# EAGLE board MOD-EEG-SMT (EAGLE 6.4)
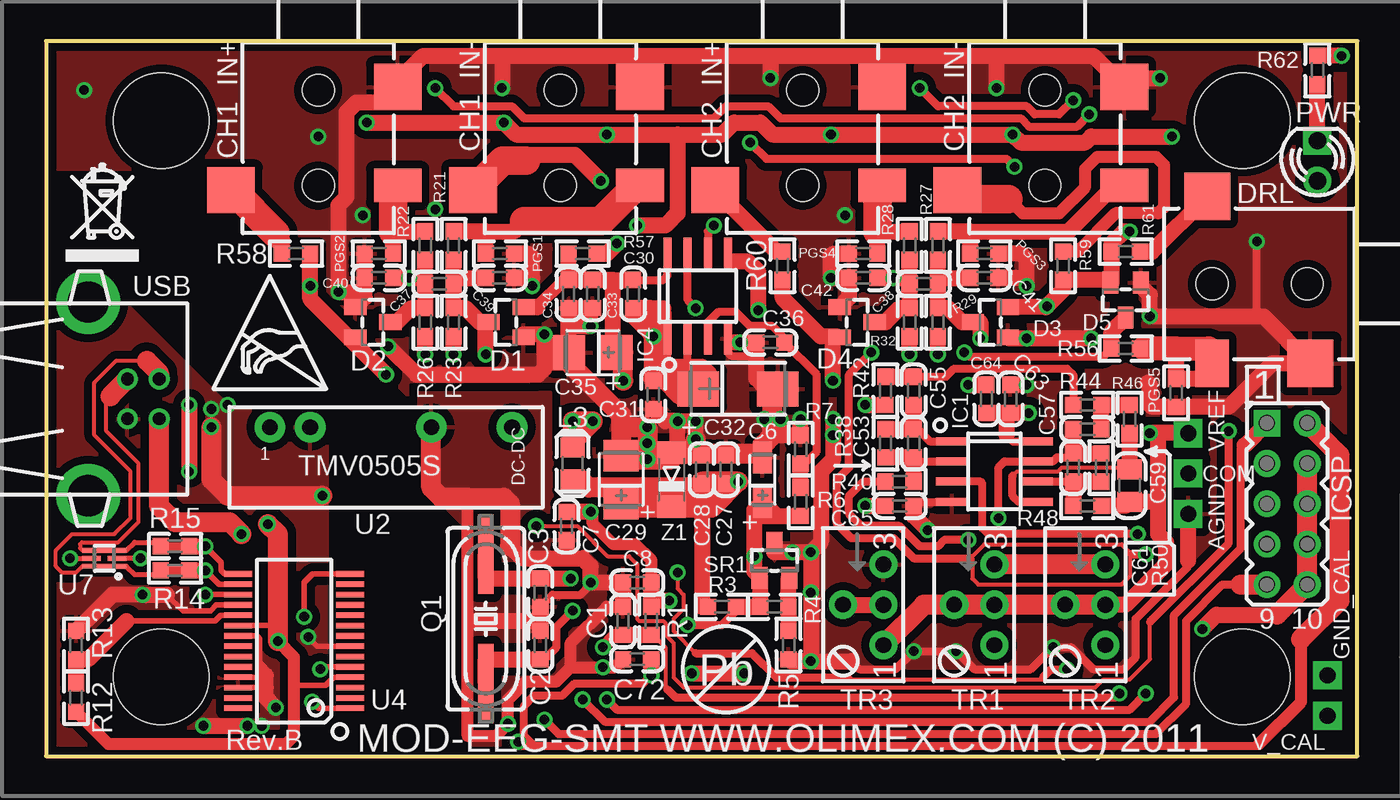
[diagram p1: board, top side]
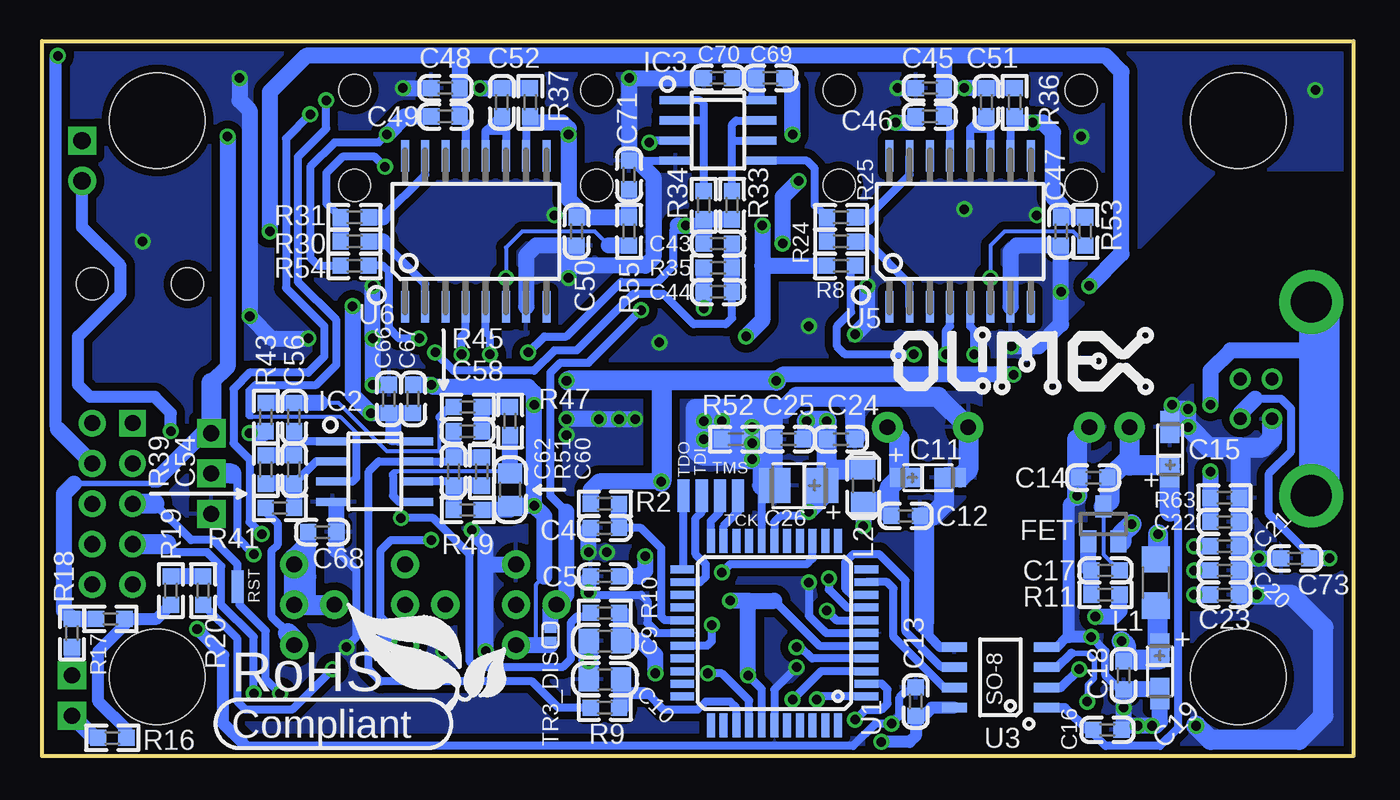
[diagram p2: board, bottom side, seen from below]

Size 82.5 x 45 mm. Coordinates in mm from the lower left corner, seen from the top.
Outline: 0,0 82.5,0 82.5,45 0,45 0,0
Copper layers (1+16): Top 0.035mm / dielectric 1.5mm / Bottom 0.035mm
Design rules "default": minimum track width 10mil, minimum drill 0.5994mm, track to track 10mil, track to pad 10mil, pad to pad 10mil, via to via 10mil, smd to smd 1mil, copper to edge 10mil, drill to drill 10mil, minimum pad ring 10mil, minimum via ring 8mil, stop-mask expansion 4mil, vias tented up to drill 25mil, thermal gap 20mil
Net classes: 1 pwr: width 0.4 mm, clearance 0.23 mm
Holes 6 mm at 7.25,5 75.25,5 7.25,40 75.25,40
tKeepout: area 22.5,43 to 30.5,45; area 21.2,0.2 to 29.2,2.2; area 45.9,0.1 to 61.9,2.1; area 45.3,43 to 61.3,45
bKeepout: area 46.8,43 to 62.8,45; area 22.5,43 to 30.5,45; area 21.2,0.2 to 29.2,2.2; area 47.3,0.2 to 63.3,2.2
tRestrict: 20 lines
bRestrict: 22 lines

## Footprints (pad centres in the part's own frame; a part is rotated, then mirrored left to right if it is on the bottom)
TEST_PAD40/70/SQUARE = drill 1.016 pad 1.778 square: P$1 0,0
C0603_DWS = smd 1.016 x 1.016: 1 -0.889,0; 2 0.889,0
CT3216 = smd 2 x 1.2: + -1.4,0; - 1.4,0
C0805_5MIL_DWS = smd 1.27 x 1.524: 1 -1.016,0; 2 1.016,0
C0603_DWS_NA = smd 1.016 x 1.016: 1 -0.889,0; 2 0.889,0
CT3528 = smd 2 x 2.2: + -1.5,0; - 1.5,0
CT6032 = smd 2.6 x 2.2: + -2.5,0; - 2.5,0
PHONE_JACK-SMD = smd 2.9 x 3: 1 -0.2,5; 5 6.3,-5.5 | smd 2.1 x 3: 2 6,5 | hole 2: 0,0; 6,0
SOT23C(BAT54S) = smd 1 x 1.4: 1 -0.95,-1.1; 2 0.95,-1.1; 3 0,1.1
SOT23 = smd 1 x 1.4: 1 -0.95,-1.1; 2 0.95,-1.1; 3 0,1.1
SO08 = smd 0.508 x 2.032: 1 -1.905,-2.667; 2 -0.635,-2.667; 3 0.635,-2.667; 4 1.905,-2.667; 5 1.905,2.667; 6 0.635,2.667; 7 -0.635,2.667; 8 -1.905,2.667
ML10_NEW = drill 1.016 pad 1.676 square: 1 -5.08,-1.27 | drill 1.016 pad 1.676: 2 -5.08,1.27; 3 -2.54,-1.27; 4 -2.54,1.27; 5 0,-1.27; 6 0,1.27; 7 2.54,-1.27; 8 2.54,1.27; 9 5.08,-1.27; 10 5.08,1.27
L1206_5MIL = smd 1.651 x 1.778: 1 -1.46,0; 2 1.46,0
L0805_5MIL_DWS = smd 1.27 x 1.524: 1 -1.016,0; 2 1.016,0
0603 = smd 1.016 x 1.016: 1 -0.889,0; 2 0.889,0
LED-3.0MM = drill 1.092 pad 1.778: A -1.27,0 | drill 1.092 pad 1.778 square: K 1.27,0
HC49/SMD2_THIN = smd 5 x 1: 1 -4.064,0; 2 4.064,0
R0603_5MIL_DWS = smd 1.016 x 1.016: 1 -0.889,0; 2 0.889,0
R0603_5MIL_DWS_NA = smd 1.016 x 1.016: 1 -0.889,0; 2 0.889,0
0603_0R = smd 1.016 x 1.016: 1 -0.889,0; 2 0.889,0
SMD80/30 = smd 2.032 x 0.762: P$1 0,0
SOT-23 = smd 1 x 1.4: 1 -0.95,-1.1; 2 0.95,-1.1; 3 0,1.1
S64Y = drill 0.991 pad 1.778: 1 2.54,1.27; 2 0,-1.27; 3 -2.54,1.27
SJ_1_SMALLER = smd 0.508 x 0.762: 1 -0.381,0; 2 0.381,0
44TQFP = smd 1.5 x 0.5: 1 -5.8,4; 2 -5.8,3.2; 3 -5.8,2.4; 4 -5.8,1.6; 5 -5.8,0.8; 6 -5.8,0; 7 -5.8,-0.8; 8 -5.8,-1.6; 9 -5.8,-2.4; 10 -5.8,-3.2; 11 -5.8,-4; 23 5.8,-4; 24 5.8,-3.2; 25 5.8,-2.4; 26 5.8,-1.6; 27 5.8,-0.8; 28 5.8,0; 29 5.8,0.8; 30 5.8,1.6; 31 5.8,2.4; 32 5.8,3.2; 33 5.8,4 | smd 0.5 x 1.5: 12 -4,-5.8; 13 -3.2,-5.8; 14 -2.4,-5.8; 15 -1.6,-5.8; 16 -0.8,-5.8; 17 0,-5.8; 18 0.8,-5.8; 19 1.6,-5.8; 20 2.4,-5.8; 21 3.2,-5.8; 22 4,-5.8; 34 4,5.8; 35 3.2,5.8; 36 2.4,5.8; 37 1.6,5.8; 38 0.8,5.8; 39 0,5.8; 40 -0.8,5.8; 41 -1.6,5.8; 42 -2.4,5.8; 43 -3.2,5.8; 44 -4,5.8
TMADCDC = drill 0.991 pad 1.93: 1 1.27,6.35; 2 1.27,3.81; 5 1.27,-3.81; 7 1.27,-8.89
SO-8_ISOLATE = smd 0.6 x 1.6: 1 -1.905,-2.9; 2 -0.635,-2.9; 3 0.635,-2.9; 4 1.905,-2.9; 5 1.905,2.9; 6 0.635,2.9; 7 -0.635,2.9; 8 -1.905,2.9
SSOP28 = smd 0.35 x 1.75: 1 -4.225,-3.525; 2 -3.575,-3.525; 3 -2.925,-3.525; 4 -2.275,-3.525; 5 -1.625,-3.525; 6 -0.975,-3.525; 7 -0.325,-3.525; 8 0.325,-3.525; 9 0.975,-3.525; 10 1.625,-3.525; 11 2.275,-3.525; 12 2.925,-3.525; 13 3.575,-3.525; 14 4.225,-3.525; 15 4.225,3.525; 16 3.575,3.525; 17 2.925,3.525; 18 2.275,3.525; 19 1.625,3.525; 20 0.975,3.525; 21 0.325,3.525; 22 -0.325,3.525; 23 -0.975,3.525; 24 -1.625,3.525; 25 -2.275,3.525; 26 -2.925,3.525; 27 -3.575,3.525; 28 -4.225,3.525
SO16 = smd 0.5 x 2: 1 -4.445,-4.75; 2 -3.175,-4.75; 3 -1.905,-4.75; 4 -0.635,-4.75; 5 0.635,-4.75; 6 1.905,-4.75; 7 3.175,-4.75; 8 4.445,-4.75; 9 4.445,4.75; 10 3.175,4.75; 11 1.905,4.75; 12 0.635,4.75; 13 -0.635,4.75; 14 -1.905,4.75; 15 -3.175,4.75; 16 -4.445,4.75
USBLC6-2P6 = smd 0.3 x 1.46: 1 -0.5,-0.65; 3 0.5,-0.65; 4 0.5,0.65; 6 -0.5,0.65 | smd 0.3 x 1.16: 2 0,-0.8; 5 0,0.8
USB_NEAR_BLACK = drill 0.8: 1 1.25,6.5; 2 -1.25,6.5; 3 -1.25,4.5; 4 1.25,4.5 | drill 2.6 pad 4: P$1 -6.096,2.032; P$2 6.096,2.032
MINI-MELF = smd 1.4 x 1.8: 1 -1.7,0; 2 1.7,0

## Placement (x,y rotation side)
AGND  TESTPAD3  [TEST_PAD40/70/SQUARE]  71.86,15.24 90 top
C1  100nF/X7R/10%  [C0603_DWS]  36.3,8.51 90 top
C2  39pF/COG/5%  [C0603_DWS]  31.09,6.99 90 top
C3  39pF/COG/5%  [C0603_DWS]  31.09,10.29 270 top
C4  10nF/X7R/10%  [C0603_DWS]  47.09,14.35 180 bottom
C5  100nF/X7R/10%  [C0603_DWS]  47.09,11.3 180 bottom
C6  10uF/6.3V/TANT  [CT3216]  45.06,17.4 90 top
C7  100nF/X7R/10%  [C0603_DWS]  32.74,14.48 270 top
C8  100nF/X7R/10%  [C0603_DWS]  37.19,10.92 180 top
C9  220nF/X7R/5%(08053C224JAT2A/1740667)  [C0805_5MIL_DWS]  47.09,7.24 180 bottom
C10  220nF/X7R/5%(08053C224JAT2A/1740667)  [C0805_5MIL_DWS]  47.09,4.83 180 bottom
C11  10uF/6.3V/TANT  [CT3216]  26.77,17.53 0 bottom
C12  100nF/X7R/10%  [C0603_DWS]  28.17,15.11 0 bottom
C13  100nF/X7R/10%  [C0603_DWS]  27.54,3.43 90 bottom
C14  100nF/X7R/10%  [C0603_DWS]  16.36,17.53 180 bottom
C15  10uF/6.3V/TANT  [CT3216]  11.53,19.3 90 bottom
C16  100nF/X7R/10%  [C0603_DWS]  15.47,1.65 0 bottom
C17  100nF/X7R/10%  [C0603_DWS]  15.6,11.68 180 bottom
C18  100nF/X7R/10%  [C0603_DWS]  14.45,5.08 270 bottom
C19  10uF/6.3V/TANT  [CT3216]  12.17,5.33 270 bottom
C20  NA  [C0603_DWS_NA]  8.1,11.68 0 bottom
C21  NA  [C0603_DWS_NA]  8.1,13.21 0 bottom
C22  10nF/X7R/10%  [C0603_DWS]  8.1,14.73 0 bottom
C23  100nF/X7R/10%  [C0603_DWS]  8.1,10.16 0 bottom
C24  10nF/X7R/10%  [C0603_DWS]  32.23,19.94 0 bottom
C25  100nF/X7R/10%  [C0603_DWS]  35.54,19.94 180 bottom
C26  47µF/6.3V/TANT  [CT3528]  34.9,17.02 180 bottom
C27  10nF/X7R/10%  [C0603_DWS]  42.77,18.03 90 top
C28  100nF/X7R/10%  [C0603_DWS]  41.25,18.03 90 top
C29  47µF/6.3V/TANT  [CT3528]  36.17,17.4 90 top
C30  100nF/X7R/10%  [C0603_DWS]  36.93,29.08 90 top
C31  100nF/X7R/10%  [C0603_DWS]  38.2,22.73 270 top
C32  47µF/10%/6.3V/TANT(C)/ESR 0.25 ohm (TR3C476K6R3C0250/1754044)  [CT6032]  43.54,23.11 0 top
C33  10nF/X7R/10%  [C0603_DWS]  34.39,29.08 270 top
C34  100nF/X7R/10%  [C0603_DWS]  32.87,29.08 270 top
C35  47µF/6.3V/TANT  [CT3528]  34.39,25.4 180 top
C36  10nF/X7R/10%  [C0603_DWS]  45.57,26.04 180 top
C37  10nF/X7R/10%  [C0603_DWS]  24.74,29.72 0 top
C38  10nF/X7R/10%  [C0603_DWS]  55.22,29.72 0 top
C39  100pF/COG/5%  [C0603_DWS]  28.55,30.1 180 top
C40  100pF/COG/5%  [C0603_DWS]  20.93,30.1 180 top
C41  100pF/COG/5%  [C0603_DWS]  59.03,30.1 180 top
C42  100pF/COG/5%  [C0603_DWS]  51.41,30.1 180 top
C43  1nF/X7R/10%  [C0603_DWS]  39.98,32.26 0 bottom
C44  1nF/X7R/10%  [C0603_DWS]  39.98,29.21 0 bottom
C45  100nF/X7R/10%  [C0603_DWS]  26.65,42.04 180 bottom
C46  100nF/X7R/10%  [C0603_DWS]  26.65,40.26 180 bottom
C47  100nF/X7R/10%  [C0603_DWS]  18.39,33.02 90 bottom
C48  100nF/X7R/10%  [C0603_DWS]  57.13,42.04 180 bottom
C49  100nF/X7R/10%  [C0603_DWS]  57.13,40.26 180 bottom
C50  100nF/X7R/10%  [C0603_DWS]  48.87,33.02 90 bottom
C51  1uF/X5R/10%  [C0603_DWS]  23.09,41.15 90 bottom
C52  1uF/X5R/10%  [C0603_DWS]  53.57,41.15 90 bottom
C53  1nF/X7R/10%  [C0603_DWS]  54.59,19.68 90 top
C54  1nF/X7R/10%  [C0603_DWS]  66.65,18.03 90 bottom
C55  1uF/X5R/10%  [C0603_DWS]  54.59,22.99 90 top
C56  1uF/X5R/10%  [C0603_DWS]  66.65,21.34 90 bottom
C57  33nF/X7R/5%(06035C333JAT2A/1740618)  [C0603_DWS]  65.51,20.57 180 top
C58  33nF/X7R/5%(06035C333JAT2A/1740618)  [C0603_DWS]  55.73,20.45 180 bottom
C59  220nF/X7R/5%(08053C224JAT2A/1740667)  [C0805_5MIL_DWS]  68.17,17.02 270 top
C60  220nF/X7R/5%(08053C224JAT2A/1740667)  [C0805_5MIL_DWS]  53.06,16.76 270 bottom
C61  1nF/X7R/10%  [C0603_DWS]  64.62,18.16 90 top
C62  1nF/X7R/10%  [C0603_DWS]  56.62,17.91 90 bottom
C63  100nF/X7R/10%  [C0603_DWS]  60.68,22.48 90 top
C64  100nF/X7R/10%  [C0603_DWS]  59.16,22.48 90 top
C65  100nF/X7R/10%  [C0603_DWS]  53.7,15.75 180 top
C66  100nF/X7R/10%  [C0603_DWS]  60.68,22.48 90 bottom
C67  100nF/X7R/10%  [C0603_DWS]  59.16,22.48 90 bottom
C68  100nF/X7R/10%  [C0603_DWS]  64.87,14.1 180 bottom
C69  100nF/X7R/10%  [C0603_DWS]  36.68,42.67 0 bottom
C70  100nF/X7R/10%  [C0603_DWS]  39.98,42.67 180 bottom
C71  100nF/X7R/10%  [C0603_DWS]  45.57,36.58 270 bottom
C72  100nF/X7R/10%  [C0603_DWS]  37.19,6.1 180 top
C73  100nF/X7R/10%  [C0603_DWS]  3.66,12.45 180 bottom
CH1_IN+  SCJ325P00XG0B02G  [PHONE_JACK-SMD]  17.12,41.91 270 top
CH1_IN-  SCJ325P00XG0B02G  [PHONE_JACK-SMD]  32.36,41.91 270 top
CH2_IN+  SCJ325P00XG0B02G  [PHONE_JACK-SMD]  47.6,41.91 270 top
CH2_IN-  SCJ325P00XG0B02G  [PHONE_JACK-SMD]  62.84,41.91 270 top
COM  TESTPAD3  [TEST_PAD40/70/SQUARE]  71.86,17.78 90 top
D1  BAV199(1156415)  [SOT23C(BAT54S)]  28.93,27.3 90 top
D2  BAV199(1156415)  [SOT23C(BAT54S)]  20.55,27.3 270 top
D3  BAV199(1156415)  [SOT23C(BAT54S)]  59.41,27.3 90 top
D4  BAV199(1156415)  [SOT23C(BAT54S)]  51.03,27.3 270 top
D5  BAV199(1156415)  [SOT23C(BAT54S)]  67.92,28.7 180 top
DRL  SCJ325P00XG0B02G  [PHONE_JACK-SMD]  79.35,29.72 180 top
FET  IRLML6402  [SOT23]  15.72,14.61 0 bottom
GND_CAL  TESTPAD3  [TEST_PAD40/70/SQUARE]  80.62,5.08 180 top
IC1  MCP607-I/SN  [SO08]  59.67,17.91 270 top
IC2  MCP607-I/SN  [SO08]  61.57,17.91 270 bottom
IC3  MCP607-I/SN  [SO08]  39.98,39.37 270 bottom
IC4  TLC277CD  [SO08]  41,28.96 0 top
ICSP  HN2x5  [ML10_NEW]  78.08,15.88 270 top
L1  FB/600 OHM/1206(321611C-601)  [L1206_5MIL]  12.42,10.92 270 bottom
L2  22µH/± 10%/1.7ohm/80mA(LB2012T220K/8030984)  [L0805_5MIL_DWS]  30.84,17.02 90 bottom
L3  22µH/± 10%/1.7ohm/80mA(LB2012T220K/8030984)  [L0805_5MIL_DWS]  33.12,18.41 270 top
PGS1  PGB1010603MR(F2594TR-ND)  [0603]  28.55,31.62 180 top
PGS2  PGB1010603MR(F2594TR-ND)  [0603]  20.93,31.62 180 top
PGS3  PGB1010603MR(F2594TR-ND)  [0603]  59.03,31.62 180 top
PGS4  PGB1010603MR(F2594TR-ND)  [0603]  51.41,31.62 180 top
PGS5  PGB1010603MR(F2594TR-ND)  [0603]  71.1,22.86 90 top
PWR  3mm_Red  [LED-3.0MM]  79.99,37.47 90 top
Q1  7.3728MHz/20pF/30ppm  [HC49/SMD2_THIN]  27.66,8.64 90 top
R1  10k  [R0603_5MIL_DWS]  38.08,8.51 270 top
R2  100R  [R0603_5MIL_DWS]  47.09,15.88 180 bottom
R3  560R  [R0603_5MIL_DWS]  42.52,9.4 180 top
R4  9.1k/1%  [R0603_5MIL_DWS]  45.82,9.4 180 top
R5  15k/1%  [R0603_5MIL_DWS]  46.71,6.99 90 top
R6  10k/1%  [R0603_5MIL_DWS]  47.47,16 270 top
R7  10k/1%  [R0603_5MIL_DWS]  47.47,19.3 270 top
R8  NA(10M)  [R0603_5MIL_DWS]  32.23,30.86 0 bottom
R9  7.5k/1%  [R0603_5MIL_DWS]  47.09,3.05 180 bottom
R10  7.5k/1%  [R0603_5MIL_DWS]  47.09,9.02 180 bottom
R11  1k  [R0603_5MIL_DWS]  15.6,10.16 180 bottom
R12  10k  [R0603_5MIL_DWS]  1.88,3.68 270 top
R13  NA  [R0603_5MIL_DWS_NA]  1.88,6.99 270 top
R14  0R(NA)  [0603_0R]  8.1,11.68 0 top
R15  0R(NA)  [0603_0R]  8.1,13.21 0 top
R16  10k/1%  [R0603_5MIL_DWS]  78.08,1.14 0 bottom
R17  100R/1%  [R0603_5MIL_DWS]  78.21,8.64 0 bottom
R18  10k/1%  [R0603_5MIL_DWS]  80.62,7.75 90 bottom
R19  1M/1%  [R0603_5MIL_DWS]  74.4,10.41 90 bottom
R20  1M/1%  [R0603_5MIL_DWS]  72.37,10.41 270 bottom
R21  2.2k/1%  [R0603_5MIL_DWS]  25.63,32.13 270 top
R22  2.2k/1%  [R0603_5MIL_DWS]  23.85,32.13 270 top
R23  2.2k/1%  [R0603_5MIL_DWS]  25.63,27.3 90 top
R24  2.2k/1%  [R0603_5MIL_DWS]  32.23,32.38 180 bottom
R25  2.2k/1%  [R0603_5MIL_DWS]  32.23,33.91 180 bottom
R26  2.2k/1%  [R0603_5MIL_DWS]  23.85,27.3 90 top
R27  2.2k/1%  [R0603_5MIL_DWS]  56.11,32.13 270 top
R28  2.2k/1%  [R0603_5MIL_DWS]  54.33,32.13 270 top
R29  2.2k/1%  [R0603_5MIL_DWS]  56.11,27.3 90 top
R30  2.2k/1%  [R0603_5MIL_DWS]  62.84,32.38 180 bottom
R31  2.2k/1%  [R0603_5MIL_DWS]  62.84,33.91 180 bottom
R32  2.2k/1%  [R0603_5MIL_DWS]  54.33,27.3 90 top
R33  10k/1%  [R0603_5MIL_DWS]  39.09,34.67 90 bottom
R34  10k/1%  [R0603_5MIL_DWS]  40.87,34.67 90 bottom
R35  200k/1%  [R0603_5MIL_DWS]  39.98,30.73 180 bottom
R36  1M/1%  [R0603_5MIL_DWS]  21.31,41.15 270 bottom
R37  1M/1%  [R0603_5MIL_DWS]  51.79,41.15 270 bottom
R38  100k/1%  [R0603_5MIL_DWS]  52.81,19.68 90 top
R39  100k/1%  [R0603_5MIL_DWS]  68.43,18.03 90 bottom
R40  1k  [R0603_5MIL_DWS]  53.7,17.27 180 top
R41  1k  [R0603_5MIL_DWS]  67.54,15.62 180 bottom
R42  1M/1%  [R0603_5MIL_DWS]  52.81,22.99 270 top
R43  1M/1%  [R0603_5MIL_DWS]  68.43,21.34 270 bottom
R44  10k/1%  [R0603_5MIL_DWS]  65.51,22.1 0 top
R45  10k/1%  [R0603_5MIL_DWS]  55.73,21.97 0 bottom
R46  15k/1%  [R0603_5MIL_DWS]  68.17,21.21 270 top
R47  15k/1%  [R0603_5MIL_DWS]  53.06,21.08 270 bottom
R48  8.2k/1%  [R0603_5MIL_DWS]  65.51,15.75 0 top
R49  8.2k/1%  [R0603_5MIL_DWS]  55.73,15.49 0 bottom
R50  100k/1%  [R0603_5MIL_DWS]  66.4,18.16 90 top
R51  100k/1%  [R0603_5MIL_DWS]  54.84,17.91 90 bottom
R52  0R(NA)  [0603_0R]  38.84,19.94 0 bottom
R53  NA(10M)  [R0603_5MIL_DWS]  16.87,33.02 270 bottom
R54  NA(10M)  [R0603_5MIL_DWS]  62.84,30.86 0 bottom
R55  NA(10M)  [R0603_5MIL_DWS]  45.57,33.02 270 bottom
R56  2.2k/1%  [R0603_5MIL_DWS]  67.92,25.65 180 top
R57  100R  [R0603_5MIL_DWS]  33.76,31.62 180 top
R58  100R  [R0603_5MIL_DWS]  15.72,31.62 0 top
R59  100R  [R0603_5MIL_DWS]  63.98,30.86 270 top
R60  100R  [R0603_5MIL_DWS]  46.33,30.86 270 top
R61  NA  [R0603_5MIL_DWS_NA]  67.92,31.75 180 top
R62  560R  [R0603_5MIL_DWS]  79.99,43.18 270 top
R63  1M  [R0603_5MIL_DWS]  8.1,16.26 180 bottom
RST  TESTPAD80/30  [SMD80/30]  70.21,10.67 90 bottom
SR1  AP431SA  [SOT-23]  45.82,12.32 0 top
TCK  TESTPAD80/30  [SMD80/30]  38.71,16.38 90 bottom
TDI  TESTPAD80/30  [SMD80/30]  41,16.38 90 bottom
TDO  TESTPAD80/30  [SMD80/30]  42.14,16.38 90 bottom
TMS  TESTPAD80/30  [SMD80/30]  39.85,16.38 270 bottom
TR1  20k  [S64Y]  58.4,9.53 270 top
TR2  20k  [S64Y]  65.38,9.53 270 top
TR3  NA(20k)???  [S64Y]  51.41,9.53 270 top
TR3_DIS  Close  [SJ_1_SMALLER]  50.52,7.62 270 bottom
U1  ATMEGA16  [44TQFP]  36.42,7.75 180 bottom
U2  TMV0505S  [TMADCDC]  20.42,19.43 90 top
U3  ISO7221XD(SOIC8)  [SO-8_ISOLATE]  22.2,4.95 90 bottom
U4  FT232RL/SSOP28  [SSOP28]  15.6,7.24 90 top
U5  INA114BU/1K  [SO16]  24.74,33.02 0 bottom
U6  INA114BU/1K  [SO16]  55.22,33.02 0 bottom
U7  NA(USBLC6-2P6)  [USBLC6-2P6]  3.66,12.45 90 top
U$1  [ESD_SYMBOL]  10.52,23.11 0 top
U$2  [OLIMEX1_V]  11.41,22.61 0 bottom
U$3  [PB]  42.77,5.46 0 top
U$4  [RECYCLE_BIN1/8]  1.25,31.11 0 top
U$11  [ROHS]  70.59,1.14 0 bottom
USB  USB_B  [USB_NEAR_BLACK]  0.61,22.48 270 top
V_CAL  TESTPAD3  [TEST_PAD40/70/SQUARE]  80.62,2.54 180 top
VREF  TESTPAD3  [TEST_PAD40/70/SQUARE]  71.86,20.32 0 top
Z1  BZV55C6V2  [MINI-MELF]  39.35,17.4 90 top

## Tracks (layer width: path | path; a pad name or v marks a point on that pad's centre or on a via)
2V_REF
  Top 0.508: IC4.3 41.63,27.3 42.27,27.94 43.41,27.94 44.3,27.05 45.7,27.05 46.46,26.29 C36.1 48.49,24 48.49,19.18 47.73,18.41 R7.2
  Top 1.016: R6.1 R7.2
4V_REF_ADC  (via drill 0.6)
  Top 0.508: v40.36,8.26 42.52,8.26 43.41,9.14 R3.1
  Top 1.016: R3.1 R4.2 44.93,11.22 SR1.1 44.87,11.3 44.55,11.62 v44.55,12.57 44.55,15.11 | 44.55,15.11 44.55,15.49 C6.+ 45.95,15.11 | 45.95,15.11 R6.2 | 44.55,15.11 45.95,15.11
  Bottom 0.508: C5.1 46.2,11.05 | U1.29 40.65,6.95 40.36,7.24 v40.36,8.26
  Bottom 0.813: 46.08,11.3 C5.1
  Bottom 1.016: v44.55,12.57 44.55,11.68 44.93,11.3 46.08,11.3
+5V  (via drill 0.6)
  Top 0.508: IC4.8 39.09,30.23 38.84,29.97 C30.2 | IC1.8 60.81,19.81 60.43,20.19 | C27.1 43.41,17.14 v43.54,17.27
  Top 0.762: C34.1 32.62,29.97 30.9,28.25
  Top 1.016: 41.25,17.02 C28.1 | R3.2 41.25,9.4 41.25,15.62 | C35.+ 35.66,25.4 35.66,29.97 | 35.66,29.97 C33.1 C34.1 R57.2 | 35.66,29.97 C30.2 | 30.9,28.25 D1.2 | 19.45,25.94 16.61,28.78 v16.61,29.59 R58.2 | D2.2 19.45,25.94 | 19.45,25.94 v21.39,24 | D3.2 62.9,28.25 v62.97,28.32 63.98,29.34 R59.2 66.97,29.97 D5.2 67.03,29.8 R61.2 67.03,32.26 67.79,33.02 v68.17,33.02 | 49.51,26.42 49.7,26.42 49.76,26.36 D4.2 | v49.51,23.62 49.51,26.42 | 49.51,26.42 48.74,26.42 46.33,28.83 R60.2 | C66.1 C67.1 | C66.1 60.43,21.59 60.43,20.19 | v61.82,21.59 C66.1
  Top 1.27: L3.2 33.63,17.4 34.14,16.89 36.17,16.89 | 36.17,16.89 36.17,16.26 | 41.25,16.89 36.17,16.89 | 36.17,16.26 C29.+ | 39.35,16.26 39.35,15.62 | 39.35,15.62 Z1.1 | 39.35,16.26 36.17,16.26 | 41.89,17.27 v43.54,17.27 41.89,15.62 | 41.89,17.27 41.25,17.27 41.25,17.02 41.25,16.89 | 41.25,16.26 39.35,16.26 | 41.25,16.89 41.25,16.26 | 41.89,15.62 41.25,15.62 | 41.25,15.62 41.25,16.26 | v36.3,23.62 36.3,25.4 C35.+ | 41.25,15.62 39.85,15.62 | 41.89,17.27 41.89,15.62 | 39.35,15.62 36.17,15.62
  Bottom 0.508: C46.1 25.38,39.88 U5.13 | 55.86,37.72 U6.13 55.86,39.88 C49.1 | IC3.8 37.57,41.27 37.57,41.53 | 60.43,20.07 60.17,19.81 IC2.8
  Bottom 1.016: R2.2 47.98,16.76 47.47,17.27 v43.54,17.27 | v36.3,23.62 35.92,24 v21.39,24 | v16.61,29.59 14.58,31.62 14.58,43.05 15.6,44.07 25.76,44.07 | 25.76,44.07 C45.1 C46.1 | C49.1 C48.1 56.24,44.07 | C69.1 37.57,41.53 | C69.1 C70.1 | 25.76,44.07 37.57,44.07 | 37.57,44.07 C69.1 | 37.57,44.07 56.24,44.07 | 56.24,44.07 65.89,44.07 68.17,41.78 v68.17,33.02 | 49.38,23.62 v49.51,23.62 | 60.43,21.59 C66.1 v61.82,21.59 62.97,22.73 v62.97,28.32 | 60.43,21.59 60.43,20.07 | 60.43,21.59 C67.1
  Bottom 1.27: 43.54,23.62 v43.54,17.27 | v36.3,23.62 43.54,23.62 | 43.54,23.62 49.38,23.62
+5V_USB
  Bottom 0.254: FET.3 15.72,12.7 C17.1
  Bottom 0.508: 11.53,15.37 11.03,14.86 11.03,1.78 12.17,0.64 15.6,0.64 16.36,1.4 C16.1
  Bottom 0.61: U3.1 18.14,3.05 16.74,1.65 C16.1
  Bottom 1.016: 15.34,17.53 C14.1
  Bottom 1.27: FET.3 15.34,16.09 15.34,17.53 14.07,18.8 | 14.07,18.8 U2.1 | 14.07,18.8 14.07,18.29 11.53,18.29 C15.+ 11.53,15.37
+12V  (via drill 0.6)
  Top 0.254: v30.84,14.48 33.43,14.48 35.33,12.57 36.68,12.57 37.19,12.06 37.19,8.64 37.31,8.51 38.84,8.51 38.96,8.38 38.96,7.62 39.47,7.11 39.47,4.95 40.11,4.32 66.02,4.32 66.52,4.83 68.17,4.83 69.44,6.1 69.44,8.43
  Top 0.508: v74.4,20.45 74.4,13.39 69.44,8.43
  Bottom 0.762: PWR.A 79.99,33.27 77.57,30.86 77.57,29.08 80.24,26.42 80.24,23.37 79.48,22.61 75.41,22.61 74.4,21.59 v74.4,20.45
  Bottom 1.016: C12.1 29.19,15.11 29.19,15.24 | L2.1 v30.84,14.48
  Bottom 1.27: U2.7 28.55,19.94 28.55,17.53 | 29.19,15.24 29.19,16 | 29.19,16 29.19,16.89 28.55,17.53 | 28.55,17.53 C11.+ | 29.19,16 L2.1
ADC0  (via drill 0.6)
  Top 1.016: v40.62,5.21 v43.92,5.21
  Bottom 0.508: C9.1 46.08,7.02 | U1.37 38.02,3.5 39.73,5.21 v40.62,5.21
  Bottom 1.016: R10.1 46.08,9.02 C9.1 44.81,7.24 43.92,6.35 v43.92,5.21
ADC1
  Bottom 0.508: 44.3,3.81 43.41,2.92 41.25,2.92 40.74,3.43 39.22,3.43 38.82,3.04 U1.36 | 44.3,3.81 44.55,4.06 46.08,4.06 | 44.3,3.81 46.08,3.81
  Bottom 1.016: R9.1 46.08,3.05 46.08,3.81 46.08,4.06 C10.1
CH1_IN+
  Top 1.016: R22.1 21.82,33.02 PGS2.1
  Top 1.778: 21.82,33.02 21.82,35.91 CH1_IN+.2
CH1_IN-
  Top 1.016: 27.66,33.02 R21.1 | 27.66,33.02 29.44,33.02 30.07,33.66 | PGS1.2 27.66,33.02
  Top 1.778: 30.07,33.66 34.9,33.66 37.16,35.91 CH1_IN-.2
CH2_IN+
  Top 1.016: R28.1 52.3,33.02 PGS4.1
  Top 1.778: 52.3,33.02 52.3,35.91 CH2_IN+.2
CH2_IN-
  Top 1.016: CH2_IN-.2 67.84,35.43 66.73,35.43 64.32,33.02 58.14,33.02 | 58.14,33.02 R27.1 | PGS3.2 58.14,33.02
DRL
  Top 1.016: DRL.2 73.35,25.65 73.13,25.65 | 69.06,25.65 R56.1 | 71.1,25.65 PGS5.2 73.25,23.75
  Top 1.524: 69.06,25.65 71.1,25.65 73.13,25.65
GND  (via drill 0.6)
  Top 0.305: 4.42,12.45 U7.2 v5.95,12.45
  Top 0.356: U4.18 10.71,9.51 10.34,9.14 8.61,9.14 7.6,10.16 | U4.7 17.06,6.91 v16.49,7.49 | U4.21 13.24,7.56 13.44,7.37 13.44,5.92 | 13.44,5.08 13.82,5.08 13.82,5.33 13.44,5.71 | 13.44,5.08 13.44,4.96 U4.25 | 13.44,5.08 13.44,5.71 | 13.44,5.71 13.44,5.92 | 13.82,4.31 U4.26 | 13.44,5.92 14.07,5.28
  Top 1.016: 7.6,10.16 v6.07,10.16 4.17,10.16 R13.1 | 13.82,5.08 13.82,4.31 13.82,3.68 v14.45,3.05 | v9.88,1.91 v12.68,1.91
  Top 1.27: v17.38,16.38 11.41,16.38 10.39,17.4 v10.39,20.7
  Bottom 0.508: C18.2 14.45,4.45 14.96,4.45 15.6,5.08 15.6,6.6 v16.49,7.49
  Bottom 0.61: 17.91,7.49 18.01,7.49 18.64,6.86 U3.4
  Bottom 0.762: 17.88,7.49 17.91,7.49 | 17.88,7.49 17.88,15.88 v17.38,16.38 | v16.49,7.49 17.88,7.49
  Bottom 1.016: C73.2 v5.95,12.45 7.09,12.45 7.09,13.21 C21.2 | 7.09,14.73 C22.2 | 7.09,10.16 C23.2 | 7.09,11.68 C20.2 | 7.09,16.26 R63.1 | 17.38,17.53 C14.2 | 11.41,20.7 11.41,20.83 10.39,20.83 v10.39,21.84 11.41,21.84 v11.41,22.1 | 14.45,1.91 v14.45,3.05 C18.2 12.17,4.19 C19.- 12.17,2.16 12.42,1.91 v12.68,1.91 v13.57,1.91 14.45,1.91 | 14.45,1.91 14.45,1.65 C16.2
  Bottom 1.27: 7.09,12.45 7.09,11.68 7.09,10.16 v6.07,10.16 3.91,10.16 1.88,8.13 1.88,2.54 3.4,1.02 8.99,1.02 v9.88,1.91 | 7.09,13.21 7.09,14.73 7.09,16.26 7.09,19.43 | USB.4 5.11,20.01 5.69,19.43 7.09,19.43 | U2.2 17.38,19.94 17.38,17.53 v17.38,16.38 | C15.- 11.41,20.7 v10.39,20.7 9.12,19.43 7.09,19.43
  pour Top (isolate 0.508, rank 3): -4.47,-1.91 -4.47,30.73 3.79,30.73 12.04,22.48 16.61,22.48 18.39,20.7 18.39,-1.91
  pour Bottom (isolate 0.508, rank 3): -4.47,-4.45 -4.47,30.73 3.79,30.73 12.04,22.48 16.61,22.48 18.39,20.7 18.39,-4.45
GNDA  (via drill 0.6)
  Top 0.508: 42.9,26.04 42.9,25.4 43.16,25.15 44.68,25.15 | 42.9,26.04 IC4.4 | IC1.4 54.84,16 C65.1 | 50.65,5.97 51.16,5.46 53.44,5.46 v54.59,6.6 v57.25,6.6 58.4,5.46 61.95,5.46 v63.35,6.86 64.49,6.86 65.89,5.46 67.79,5.46 68.56,6.22 68.56,8.64 71.86,11.94 71.86,12.29 | 76.18,27.69 v76.18,32.38 | 43.16,26.04 42.9,26.04
  Top 1.016: 41.25,19.05 C28.2 | 42.77,19.05 C27.2 | 39.73,19.05 v39.73,21.08 | v40.87,19.94 v40.87,21.08 v39.73,21.08 | SR1.3 45.82,12.83 v46.97,12.83 v48.11,12.83 | v48.11,5.97 46.84,5.97 R5.1 | 32.87,25.4 C35.- | 32.87,25.4 32.87,25.91 | 32.87,25.91 32.87,27.05 | 32.87,27.05 C34.2 C33.2 34.27,28.19 v34.27,27.05 32.87,27.05 | 30.58,30.1 C39.1 | D1.1 30.03,26.54 v31.34,26.54 31.34,25.91 | 32.87,25.4 32.87,24.77 31.34,24.77 | 31.34,24.77 31.34,24.38 30.96,24 23.29,24 v21.52,25.78 | 31.34,24.77 31.34,25.4 | 31.34,25.4 31.34,25.91 | CH1_IN+.1 22.12,42.08 21.18,41.15 19.53,41.15 18.9,40.51 18.9,35.18 18.39,34.67 v18.39,29.21 19.35,29.21 19.35,28.25 D2.1 20.04,28.85 C40.2 PGS2.2 | CH1_IN+.1 22.12,42.04 | CH1_IN+.1 22.12,42.47 23.72,44.07 28.68,44.07 | 61.7,30.1 C41.1 | D3.1 60.58,26.29 v61.7,26.29 v65.76,26.29 | 52.6,42.04 CH2_IN+.1 52.6,44.07 | 28.68,44.07 v28.68,42.04 | 28.68,44.07 37.36,44.07 | 45.57,44.07 52.6,44.07 | 59.79,44.07 65.88,44.07 CH2_IN-.1 67.84,42.67 v70.08,42.67 | 37.36,44.07 CH1_IN-.1 | 37.36,44.07 45.57,44.07 | 59.79,44.07 v59.79,42.04 | 52.6,44.07 59.79,44.07 | D5.1 68.87,29.59 69.44,29.02 v69.44,27.69 76.18,27.69 76.58,27.69 DRL.1 77.14,24.72 74.4,21.97 PGS5.1 69.57,21.97 69.44,22.1 69.44,23.37 69.32,23.5 | 46.2,20.19 R7.1 v47.47,21.21 | 49.93,28.32 D4.1 50.52,28.85 C42.2 v49.38,30.1 49.38,31.5 49.51,31.62 PGS4.2 | 45.57,44.07 v45.57,42.67 | 45.7,23.11 45.31,23.11 44.68,23.75 44.68,25.15 C36.2 v43.66,26.04 43.16,26.04 | C31.2 38.96,21.08 v39.73,21.08 | v48.11,5.97 v48.11,10.29 v48.11,12.83 | v61.7,23.37 C66.2 | v48.11,5.97 50.65,5.97 | 71.86,12.29 AGND.P$1 | v55.48,14.22 54.59,15.11 C65.1 | PGS1.1 30.33,31.62 30.58,31.37 30.58,30.1
  Top 1.016: v30.58,29.59 30.58,30.1 | PGS3.1 61.32,31.62 61.7,31.24 61.7,30.1 | v61.7,29.59 61.7,30.1 | v48.11,12.83 48.74,13.46 48.74,17.91 49.51,18.67 v49.51,20.19 v49.51,21.21 | 45.7,20.19 46.2,20.19 | 46.2,20.19 v46.2,21.21 | 31.34,25.91 32.87,25.91 | 31.34,25.4 32.87,25.4
  Top 1.27: 39.35,19.05 39.35,18.67 v37.82,18.67 | 39.35,19.05 Z1.2 | 39.35,19.05 39.73,19.05 40.87,19.05 | 40.87,19.05 41.25,19.05 42.77,19.05 45.06,19.05 | 40.87,19.05 v40.87,19.94 | 45.06,19.05 C6.- | 36.17,20.7 36.17,21.46 32.89,24.74 C35.- | 36.17,20.7 C29.- 36.17,18.67 v37.82,18.67 | 45.06,19.05 45.06,19.56 45.7,20.19 45.7,23.11 C32.- | 36.17,20.7 v37.82,20.7 v37.82,19.68 v37.82,18.67
  Bottom 0.508: 47.98,11.18 C5.2 | C71.1 IC3.4 | IC2.4 63.98,16 63.98,15.75 | v63.35,6.86 62.71,7.49 62.71,11.68 63.98,12.95 | U1.28 43.79,7.75 44.43,8.38 44.43,9.78 44.81,10.16 48.11,10.16 v48.11,10.29
  Bottom 1.016: v31.34,26.54 30.58,27.3 v30.58,29.59 | v21.52,25.78 19.79,25.78 18.39,27.18 v18.39,29.21 C47.1 21.18,32.13 21.57,31.75 U5.7 | v28.68,42.04 C45.2 | v61.7,29.59 v61.7,26.29 v61.7,23.37 C66.2 | v59.79,42.04 C48.2 | U6.7 52.05,31.5 51.41,32.13 49.38,32.13 | 49.38,32.13 C50.1 48.87,30.86 44.55,30.86 44.05,31.37 44.05,36.45 45.06,37.47 C71.1 v45.57,42.67 C70.2 | 49.38,32.13 v49.38,30.1 | v70.08,42.67 70.08,41.27 69.44,40.64 v69.44,27.69 68.05,26.29 v65.76,26.29 | 63.98,15.75 C68.1 63.98,12.95 | 54.59,12.06 54.59,13.34 v55.48,14.22 | v45.19,21.21 v47.47,21.21 v49.51,21.21 | 54.59,12.06 TR3.3 | v54.59,6.6 54.59,12.06 | 47.98,11.18 48.11,11.18 v48.11,10.29 | C4.2 48.11,14.35 v48.11,12.83
  Bottom 1.27: C10.2 v48.11,5.97 C9.2 | v39.73,21.08 R52.1 v40.87,19.94 v40.87,21.08 v39.73,21.08
  other vias: 2.39,41.91 17.12,38.99 50.27,34.04 24.49,34.42 19.91,34.04
  pour Top (isolate 0.508, rank 2): -2.56,36.2 8.23,36.2 23.47,20.95 23.47,16.51 26.01,13.97 26.01,-5.08 88.24,-5.08 88.24,46.99 -2.56,46.99
  pour Bottom (isolate 0.508, rank 2): -2.56,36.2 8.23,36.2 23.47,20.95 23.47,16.51 26.01,13.97 26.01,-5.08 85.7,-5.08 85.7,46.99 -2.56,46.99
MISO  (via drill 0.6)
  Top 0.508: 75.16,10.79 74.02,10.79 71.73,8.51 71.73,3.3 69.83,1.4 32.23,1.4 v31.34,2.29
  Top 1.27: 75.16,10.79 ICSP.9
  Bottom 0.508: v31.34,2.29 30.71,2.92 29.69,2.92 29.31,3.3 29.31,4.19 29.67,4.55 U1.2
MOSI  (via drill 0.6)
  Top 0.508: 75.41,19.56 75.16,19.3 75.16,13.06 70.97,8.87 70.97,3.68 69.44,2.16 35.16,2.16 v33.76,3.56
  Top 1.016: 75.41,19.56 ICSP.1
  Bottom 0.508: v33.76,3.56 33.57,3.75 U1.1
N$1
  Top 0.305: U7.1 5.05,11.95 5.56,11.43 7.21,11.43 R14.1
N$2
  Top 0.305: U7.3 5.05,12.95 5.56,13.46 7.21,13.46 R15.1
N$3
  Bottom 0.508: U1.24 41.1,10.95 40.74,11.3 40.74,12.06 41.38,12.7 41.38,14.99 41,15.37 TDI.P$1
N$4
  Bottom 0.508: U1.23 42.14,11.75 TDO.P$1
N$5
  Bottom 0.508: U1.22 40.42,14.8 39.85,15.37 TMS.P$1
N$6
  Bottom 0.508: U1.21 39.62,14.48 38.71,15.39 TCK.P$1
N$7  (via drill 0.6)
  Top 1.016: 30.2,37.47 30.58,37.85 33.25,37.85 v34.9,36.2 | v35.92,32.26 35.28,31.62 R57.1
  Top 1.778: CH1_IN-.5 28.72,37.47 30.2,37.47
  Bottom 1.016: v34.9,36.2 35.92,35.18 v35.92,32.26
N$8
  Top 1.016: R58.1 14.84,32.51 14.45,32.89
  Top 1.778: CH1_IN+.5 11.74,35.61 14.45,32.89
N$9  (via drill 0.6)
  Top 0.508: v57.76,25.4 58.02,25.15 66.52,25.15 R56.2
  Top 1.016: D5.3 67.03,26.71 R56.2
  Bottom 0.508: C44.2 39.09,27.56 39.47,27.18 41.51,27.18 43.41,29.08 45.31,29.08 48.87,25.53 50.27,25.53 51.54,24.26 56.62,24.26 v57.76,25.4
  Bottom 1.016: C43.2 R35.1 C44.2
N$10
  Top 1.016: CH2_IN+.5 43.04,34.67 43.03,34.67 45.95,31.75 R60.1
N$11
  Top 0.762: 60.55,35.05 61.44,34.16 63.73,34.16 65.38,35.81 65.38,36.96 66.14,37.72 69.83,37.72 70.33,37.21 70.33,34.54 69.95,34.16 67.29,34.16 64.87,31.75 R59.1
  Top 1.778: CH2_IN-.5 57.34,35.05 60.55,35.05
N$12
  Top 1.016: DRL.5 69.58,31.75 R61.1
N$15
  Top 1.016: PWR.K R62.2
N$16  (via drill 0.6)
  Top 0.356: v17.25,5.46 17.4,5.61 U4.5
  Bottom 0.61: U3.2 18.39,4.32 v17.25,5.46
N$17  (via drill 0.6)
  Top 1.016: v8.99,22.1 v8.99,17.91
  Bottom 1.016: C22.1 R63.2 v8.99,17.91 | v8.99,22.1 8.99,24.26 7.72,25.53 2.13,25.53
  Bottom 2.54: USB.P$2 2.13,16.89 2.13,25.53 2.13,28.07 USB.P$1
N$18
  Top 0.254: U7.6 2.27,11.95 1.88,11.56 0.99,11.56 0.61,11.94 0.61,12.95 1.63,13.97 4.29,13.97 5.31,14.99 5.31,17.91 3.02,20.19 3.02,23.5 4.42,24.89 6.33,24.89
  Top 1.27: 6.33,24.89 7.11,24.11 USB.2
N$20  (via drill 0.6)
  Top 0.356: U4.1 17.15,3.01 v16.74,3.43
  Bottom 0.356: v16.74,3.43 16.74,4.45 16.28,4.9 16.28,6.02 16.74,6.48 17.76,6.48
  Bottom 0.61: U3.3 18.64,5.59 17.76,6.48
N$21
  Bottom 0.508: U1.27 43.32,8.55 43.54,8.76 43.54,13.08 44.81,14.35 C4.1
  Bottom 1.016: C4.1 R2.1
N$22
  Top 1.016: SR1.2 46.71,11.22 R4.1 R5.2
N$23
  Bottom 0.508: U1.10 29.34,10.95 28.93,10.54 28.93,7.49 25.76,4.32 U3.7
N$24
  Bottom 0.508: U1.9 31.56,10.15 31.98,10.57 31.98,12.19 31.47,12.7 29.82,12.7 28.17,11.05 28.17,7.85 25.91,5.59 U3.6
N$25
  Top 0.254: U7.4 2.27,12.95 2.13,13.08 2.13,13.34 2.26,13.46 4.55,13.46 5.82,14.73 5.82,18.41 3.79,20.45 3.79,22.4 4.04,22.66
  Top 1.27: 4.04,22.66 USB.3
N$26  (via drill 0.6)
  Top 0.305: v1.5,12.45 U7.5
  Top 1.27: USB.1 7.09,21.23 7.09,15.75 8.1,14.73 11.53,14.73 v12.3,13.97
  Bottom 0.508: 6.2,22.48 4.55,22.48 3.91,21.84 3.91,19.18 5.31,17.78 5.31,15.24 2.77,12.7 C73.1
  Bottom 1.016: v1.5,12.45 C73.1 | USB.1 7.11,21.57 6.2,22.48
  Bottom 1.27: v12.3,13.97 12.3,12.38 L1.1
N$27  (via drill 0.6)
  Top 0.508: C3.1 30.07,11.18
  Top 1.016: Q1.2 27.66,11.18 C3.1 v33,11.18
  Bottom 0.508: U1.8 31.85,9.35 33,10.49 v33,11.18
N$28  (via drill 0.6)
  Top 0.508: C2.1 31.34,6.1 32.11,6.86 32.11,8.13 v33.12,9.14
  Top 1.016: Q1.1 27.66,6.1 C2.1
  Bottom 0.508: v33.12,9.14 32.53,8.55 U1.7
N$29  (via drill 0.6)
  Top 0.508: R40.2 51.41,17.27 50.52,16.38 50.52,15.24 51.28,14.48 53.7,14.48 54.97,13.21 56.11,13.21 56.49,13.59 v58.02,13.59
  Bottom 0.508: 60.81,7.87 61.19,8.26 61.19,8.76 | 61.19,8.76 61.19,12.95 60.55,13.59 v58.02,13.59 | 61.19,8.76 60.55,8.13
  Bottom 1.27: TR1.1 59.92,6.99 60.81,7.87
N$30
  Bottom 0.508: 67.03,7.75 68.05,8.76 68.05,12.95 67.67,13.34 67.67,14.61 68.43,15.37 R41.2
  Bottom 1.27: TR2.1 66.65,7.37 67.03,7.75
N$35
  Top 0.356: U4.19 10.97,8.86 10.62,8.51 5.06,8.51
  Top 1.016: 5.06,8.51 2.64,6.1 R13.2 R12.1
N$78  (via drill 0.6)
  Top 0.356: U4.17 v10.01,10.16
  Bottom 1.016: C23.1 v10.01,10.16
N$79  (via drill 0.6)
  Top 0.356: 14.58,8.21 U4.20 | 15.6,4.45 17.58,4.45 18.1,4.96 U4.4
  Top 0.762: v14.58,7.24 15.6,6.22 15.6,4.45 15.6,1.27 15.09,0.76 3.91,0.76 R12.2
  Top 1.27: v14.58,7.24 14.58,8.21 14.58,13.97 v13.95,14.61
  Bottom 0.762: 14.58,13.53 14.58,13.51 FET.2
  Bottom 1.016: C18.1 14.33,6.1 14.2,6.1
  Bottom 1.27: v14.58,7.24 14.33,6.99 14.33,6.1 | L1.2 12.3,9.46 12.3,6.73 C19.+ 12.17,6.1 14.2,6.1 | v13.95,14.61 14.58,13.97 14.58,13.53
N$81
  Top 0.508: C55.2 56.62,23.88 57.13,24.38 64.24,24.38 64.62,24 R44.1
  Top 1.016: R42.1 C55.2
N$83
  Bottom 0.508: 22.84,39.88 22.84,40.01 C51.1 23.34,40.26 23.72,39.88 | 22.84,39.5 22.84,39.88 | 22.84,39.5 U5.11 | U5.12 24.11,39.5 | 24.11,39.5 23.72,39.88 | 23.72,39.88 22.84,39.88 | 24.11,39.5 22.84,39.5
N$84  (via drill 0.6)
  Top 1.016: v25.63,25.27 R23.1
  Bottom 0.508: v25.63,25.27 25.63,26.8 25.38,27.05 U5.4
N$88
  Bottom 0.508: U5.2 27.92,29.72 30.58,32.38
  Bottom 1.016: 30.58,32.38 R24.1
N$92  (via drill 0.6)
  Top 1.016: 23.85,30.1 R22.2 | 23.85,30.1 C37.1 R26.2 22.96,28.19 22.07,27.3 D2.3 | 23.85,30.1 v22.84,30.1 C40.1
  Bottom 0.254: R53.2 16.87,32.26 17.63,33.02 21.95,33.02 22.84,32.13 v22.84,30.1
N$93  (via drill 0.6)
  Top 1.016: 25.63,30.1 R21.2 | 25.63,30.1 C37.2 R23.2 26.39,28.19 27.28,27.3 27.66,27.3 | 25.63,30.1 C39.2 | 27.66,27.3 D1.3 | v27.66,25.27 27.66,27.3
  Bottom 0.508: R8.2 31.6,30.61 31.6,27.94 32.49,27.05 32.49,25.78 31.98,25.27 v27.66,25.27
N$94  (via drill 0.6)
  Top 1.016: 54.33,30.1 v53.32,30.1 C42.1 | 54.33,30.1 C38.1 R32.2 53.7,28.19 52.81,27.3 D4.3 | 54.33,30.1 R28.2
  Bottom 0.254: 46.84,32.13 47.73,33.02 52.3,33.02 53.32,32 v53.32,30.1
  Bottom 1.016: R55.2 46.84,32.13
N$95  (via drill 0.6)
  Top 0.508: D3.3 58.27,27.3
  Top 1.016: 56.11,30.1 R27.2 | 56.11,30.1 C38.2 R29.2 56.74,28.19 57.63,27.3 D3.3 58.78,27.3 v58.78,26.29 | 56.11,30.1 C41.2
  Bottom 0.508: R54.2 61.06,30.86 60.68,30.48 60.68,26.92 60.05,26.29 v58.78,26.29
N$101
  Bottom 0.508: U5.15 27.92,36.58 30.58,33.91
  Bottom 1.016: R25.1 30.58,33.91
N$102  (via drill 0.6)
  Top 0.508: v24.49,42.04 25.63,40.89 29.31,40.89 30.07,40.13 42.01,40.13 42.77,40.89 45.44,40.89 46.2,40.13 61.32,40.13 61.82,39.62 64.87,39.62 v65.64,40.39 | IC1.3 58.78,17.27 58.9,17.14 58.9,14.35 59.28,13.97 v68.68,13.97
  Bottom 0.508: v65.64,40.39 67.16,38.86 67.16,29.46 64.75,27.05 64.75,25.15 65.76,24.13 69.44,24.13 70.46,23.11 70.46,19.68 69.44,18.67 69.44,14.73 v68.68,13.97
  Bottom 1.016: R36.1 C51.2 v24.49,42.04
N$103
  Bottom 0.508: IC3.5 34.39,37.47 33.88,36.96 33.88,34.67 R25.2
  Bottom 1.016: R24.2 R25.2
N$104
  Top 0.508: C53.2 54.84,20.57 55.6,19.81 IC1.1
  Top 1.016: C55.1 C53.2 R38.2
N$105
  Top 0.508: 54.59,18.54 IC1.2
  Top 1.016: R38.1 C53.1 54.59,18.54 R40.1
N$106  (via drill 0.6)
  Top 1.016: v23.85,25.27 R26.1
  Bottom 0.508: v23.85,25.27 23.85,26.8 24.11,27.05 U5.5
N$107
  Top 0.254: C59.1 68.17,18.16 63.91,18.16 63.65,17.91 61.06,17.91 60.81,17.65
  Top 0.508: 60.81,17.65 60.81,16.38 61.19,16 IC1.5
  Top 1.016: C59.1 R46.2
N$108
  Top 1.016: R46.1 R44.2 C57.1
N$109  (via drill 0.6)
  Top 0.508: C61.2 64.36,18.8 63.6,18.8 63.35,18.54 IC1.7 60.3,18.54 59.92,18.16 v59.92,14.99
  Top 1.016: C57.2 C61.2 R50.2
  Bottom 0.508: v59.92,14.99 57.89,14.99 55.6,12.7 55.6,5.97 55.22,5.59 49.76,5.59 49.25,6.1 49.25,8.38 48.87,8.76 48.24,8.76 R10.2
N$110
  Top 0.508: IC1.6 C61.1
  Top 1.016: R50.1 C61.1 R48.1
N$113  (via drill 0.6)
  Top 0.508: v54.97,42.04 56.11,40.89 61.7,40.89 62.21,40.39 63.73,40.39 v64.62,41.27
  Bottom 0.254: 69.44,21.46 69.32,21.34 63.73,21.34 62.71,20.32 62.71,20.14
  Bottom 0.508: v64.62,41.27 64.62,39.5 66.4,37.72 66.4,29.84 63.98,27.43 63.98,24.64 65.25,23.37 69.06,23.37 69.44,22.99 69.44,21.46 | IC2.3 62.97,17.27 62.71,17.53 62.71,20.14
  Bottom 1.016: C52.2 R37.1 v54.97,42.04
N$125
  Bottom 0.508: IC2.1 66.65,19.81
  Bottom 1.016: C56.1 66.65,19.81 C54.2 R39.2
N$126
  Bottom 0.508: IC2.2 65.25,18.54 C54.1
  Bottom 1.016: R39.1 C54.1 R41.1
N$127
  Bottom 0.254: 60.17,17.91 60.43,17.65 | C60.1 53.06,17.91 60.17,17.91 | 60.55,17.65 60.55,17.78 60.43,17.91 60.17,17.91
  Bottom 0.508: IC2.5 60.05,16 60.43,16.38 60.43,17.65
  Bottom 1.016: C60.1 R47.2
N$128
  Bottom 1.016: R47.1 R45.2 C58.1
N$129
  Bottom 0.508: R9.2 50.01,3.05 51.66,4.7 61.19,4.7 61.95,5.46 61.95,17.91 61.32,18.54 IC2.7 56.87,18.54 C62.2
  Bottom 1.016: C58.2 C62.2 R51.2
N$130
  Bottom 0.508: C62.1 56.62,17.27 IC2.6
  Bottom 1.016: R51.1 C62.1 R49.1
N$131
  Bottom 0.254: 57.51,21.34 57.51,19.3 57.63,19.18 60.81,19.18 63.86,22.23 65,22.23
  Bottom 0.508: R45.1 56.87,21.97 57.51,21.34
  Bottom 1.016: R43.1 C56.2 65,22.23
N$133
  Bottom 0.508: 53.32,39.37 53.32,39.75 | 53.32,39.75 53.32,40.26 C52.1 53.7,40.26 54.2,39.75 | 53.32,39.37 U6.11 | U6.12 54.59,39.37 | 54.59,39.37 54.2,39.75 | 54.59,39.37 53.32,39.37 | 54.2,39.75 53.32,39.75
N$134
  Bottom 0.508: U6.2 58.4,29.72 61.06,32.38
  Bottom 1.016: 61.06,32.38 R30.1
N$135
  Bottom 0.508: U6.15 58.4,36.58 61.06,33.91
  Bottom 1.016: R31.1 61.06,33.91
N$136  (via drill 0.6)
  Top 0.508: v44.3,38.61 45.31,37.59 60.43,37.59 v60.94,37.08
  Bottom 0.508: IC3.3 44.17,38.73 v44.3,38.61 | v60.94,37.08 61.57,37.72 63.6,37.72 64.62,36.7 64.62,34.8 R31.2
  Bottom 1.016: R31.2 R30.2
N$137  (via drill 0.6)
  Top 1.016: v56.11,25.27 R29.1
  Bottom 0.508: v56.11,25.27 R29.1 55.86,26.67 U6.4
N$138  (via drill 0.6)
  Top 1.016: v54.33,25.27 R32.1
  Bottom 0.508: v54.33,25.27 R32.1 54.59,26.67 U6.5
N$139
  Bottom 0.508: 40.87,40.01 IC3.2 | R34.2 40.87,40.01 | IC3.1 41.12,41.27 40.87,41.02 40.87,40.01
N$140
  Bottom 0.508: IC3.7 38.84,40.01 39.09,39.75 39.09,38.73 | 39.09,38.73 IC3.6 | R33.2 39.09,38.73
N$141  (via drill 0.6, 1 pad 1.78)
  Top 0.508: 43.16,31.11 42.9,31.11 IC4.5
  Top 1.016: v44.81,28.07 44.81,30.48 44.17,31.11 43.16,31.11 | TR3.2 v52.68,9.53
  Bottom 0.508: v44.81,28.07 48.11,24.77 49.89,24.77 50.52,24.13 50.52,16.38 49.51,15.37 | TR3_DIS.1 50.52,8.26
  Bottom 1.016: 49.51,15.37 49.51,10.16 TR3.2 50.52,9.14 50.52,8.26
N$142  (via drill 0.6)
  Top 0.508: IC4.7 40.36,28.7 v40.87,28.19
  Bottom 1.016: R35.2 C44.1 v40.87,28.19
N$144
  Bottom 1.016: R20.1 R19.2
N$145  (via drill 0.6)
  Top 0.254: 58.14,12.45 59.03,13.34 67.67,13.34 68.3,12.7 68.17,12.7 68.17,11.3 67.67,10.79 58.65,10.79 58.27,11.18 58.27,12.45 58.14,12.45
  Top 0.508: v42.01,33.4 41.63,33.02 IC4.6 | v51.92,25.4 50.52,24 50.52,18.16 49.76,17.4 49.76,14.61 50.65,13.72 53.32,13.72 54.59,12.45 58.14,12.45 | 68.3,12.7 v69.19,12.7
  Bottom 0.508: 42.52,33.4 42.77,33.15 42.77,30.86 43.79,29.84 46.08,29.84 49.51,26.42 50.9,26.42 v51.92,25.4 | v69.19,12.7 70.21,13.72 70.21,17.78 70.59,17.78
  Bottom 1.016: R33.1 R34.1 40.87,33.4 | 40.87,33.4 v42.01,33.4 42.52,33.4 | 40.87,33.4 C43.1
  Bottom 1.27: 70.59,17.78 COM.P$1
N$146
  Bottom 0.762: R16.2 77.19,1.65 78.97,3.43 78.97,6.6 77.32,8.26 R17.2 75.29,8.64 R19.1
N$148
  Bottom 1.016: V_CAL.P$1 79.22,1.14 R16.1
N$149
  Bottom 1.016: GND_CAL.P$1 R18.1
N$168
  Bottom 1.016: FET.1 16.67,11.87 C17.2 R11.2
PD5  (via drill 0.6)
  Top 0.254: v39.73,11.56 39.73,10.54 40.11,10.16 40.11,9.27 39.47,8.64 39.47,7.87 40.87,6.48 | 50.39,4.95 50.52,4.83 50.7,4.83 | 50.7,4.83 62.59,4.83 62.71,4.95 | 50.7,4.83 50.57,4.95
  Top 0.508: 40.87,6.48 44.43,6.48 45.95,4.95 50.39,4.95 | 62.71,4.95 63.22,5.46 v64.24,5.46
  Bottom 0.508: R20.2 70.21,7.37 70.21,3.43 69.7,2.92 66.78,2.92 v64.24,5.46 | U1.14 34.02,12.43 34.39,12.06 39.22,12.06 v39.73,11.56
PE  (via drill 0.6)
  Top 0.508: 31.09,9.53 C3.2 31.85,10.16 33.63,10.16 34.27,10.79 v34.27,10.92 | 29.19,13.21 28.8,13.21
  Top 0.762: 26.52,8.51 26.52,16.26 | 26.52,8.51 26.52,1.27 28.3,1.27 v29.06,2.03 29.06,3.56 30.2,4.7 32.11,4.7 33,5.59 | 26.52,8.51 26.65,8.51 | C72.2 35.79,5.59 v35.03,5.59 33,5.59 | 33,5.59 33,7.11 35.28,9.4 C1.2
  Top 1.016: 31.09,8.51 C2.2 | 31.09,8.51 C3.2 | 26.65,8.51 31.09,8.51 | v72.75,8 73.64,8.89 77.45,8.89 | v81.51,44.07 R62.1 | C1.2 C8.2 v34.27,10.92 34.27,11.94 33.76,12.45 32.74,12.45 | 32.74,12.45 29.95,12.45 29.19,13.21 | 32.74,12.45 C7.2
  Top 1.27: U2.5 24.23,16.89 24.87,16.26 26.52,16.26 28.8,16.26 29.19,15.88 29.19,13.21 | 77.45,8.89 ICSP.10 ICSP.8 ICSP.6 ICSP.4
  Bottom 0.508: U1.6 33.17,7.75 34.27,8.84 v34.27,10.92 | U1.39 36.42,4.19 v35.03,5.59 | U1.18 37.23,16.98 37.19,17.02 | 69.83,0.76 69.7,0.64 31.47,0.64 30.07,2.03 v29.06,2.03 28.55,2.54 28.55,3.68 28.17,4.06 27.79,4.06 C13.2 | 26.65,7.49 26.65,8.33
  Bottom 0.61: 27.03,8.33 27.03,7.87 26.65,7.49 26.01,6.86 U3.5
  Bottom 0.762: 27.03,15.11 C12.2 | 69.83,0.76 71.1,2.03 71.1,6.35 v72.75,8 | 81.51,20.57 81.64,20.7 81.64,43.94 v81.51,44.07
  Bottom 1.016: 26.52,15.11 27.03,15.11 | 36.55,19.94 C25.2 | 31.34,20.07 C24.2 | ICSP.4 81.51,20.57
  Bottom 1.27: 26.52,15.11 25.76,15.88 25.76,17.53 C11.- 24.74,17.53 24.23,18.03 U2.5 26.14,22.61 31.34,22.61 | 27.03,15.11 27.03,8.33 | 36.55,21.84 36.55,20.83 | 36.55,20.83 36.55,19.94 | 36.55,17.02 C26.- | 36.55,19.94 36.55,18.03 | 36.55,18.03 36.55,17.02 | 31.34,22.61 31.34,20.07 | 31.34,22.61 35.03,22.61 35.79,21.84 36.55,21.84 | 36.55,19.94 R52.2 | 39.47,19.94 38.46,19.94 37.19,18.67 | 39.47,19.94 39.73,20.19 39.73,18.92 41,18.92 41.38,19.3 41.38,20.83 | 36.55,21.84 41.38,21.84 41.38,20.83 | 36.55,18.03 37.19,18.67 | 36.55,17.02 37.19,17.02 37.19,18.67 | 37.19,18.67 38.71,18.67 39.47,19.43 39.47,19.94 | 36.55,20.83 41.38,20.83
  pour Bottom (isolate 0.508): 23.47,23.5 23.47,-6.99 39.35,-6.99 39.35,3.17 43.16,3.17 43.16,23.5
  pour Top (isolate 0.508): 23.47,22.86 23.47,-8.26 39.35,-8.26 39.35,3.17 43.16,3.17 43.16,19.05 31.73,19.05 31.73,22.86
PWREN  (via drill 0.6)
  Top 0.356: U4.14 16.77,11.46 16.23,10.92 v16.23,8.76
  Bottom 1.016: v16.23,8.76 15.09,8.76 14.71,9.14 R11.1
RST  (via drill 0.6)
  Top 0.254: 38.2,7.62 38.96,6.86 38.96,4.32 39.09,4.19
  Top 0.508: R1.2 38.2,7.62 | 39.09,4.19 39.6,3.68 67.29,3.68 v67.54,3.94
  Top 0.762: C1.1 35.79,7.62 v35.03,6.86
  Top 1.016: C1.1 R1.2
  Bottom 0.508: 75.44,15.88 75.41,15.88 73.13,13.59 71.73,13.59 70.21,12.06 RST.P$1 70.21,10.29 70.08,10.16 70.08,9.53 68.43,7.87 68.43,4.83 v67.54,3.94 | U1.4 34.06,6.15 34.77,6.86 v35.03,6.86
  Bottom 1.27: 75.44,15.88 ICSP.5
SCK  (via drill 0.6)
  Top 0.508: v69.19,3.94 68.17,2.92 35.92,2.92 v35.28,3.56
  Bottom 0.508: v69.19,3.94 69.19,7.49 71.22,9.53 71.22,11.94 72.11,12.83 74.14,12.83 74.65,13.34 74.68,13.34 | U1.3 33.49,5.35 v35.28,3.56
  Bottom 1.27: 74.68,13.34 ICSP.7
USBDM  (via drill 0.6)
  Top 0.356: U4.16 10.88,10.81 v10.01,11.68
  Top 1.016: R14.2 v10.01,11.68
  Bottom 1.016: v10.01,11.68 R14.2
USBDP  (via drill 0.6)
  Top 0.356: U4.15 11.25,11.46 11.03,11.68 11.03,12.19 v10.01,13.21
  Top 1.016: R15.2 v10.01,13.21
  Bottom 1.016: v10.01,13.21 R15.2
VCC/2  (via drill 0.6, 1 pad 1.78)
  Top 0.508: 38.84,28.19 39.09,27.94 IC4.1 39.09,24.51 39.09,23.62 | 40.36,23.62 40.36,24.51 IC4.2 | 40.36,23.11 C32.+
  Top 1.016: v20.17,39.88 v28.8,39.88 29.57,39.12 v35.28,39.12 39.73,39.12 | 39.73,39.12 42.52,39.12 43.28,39.88 44.93,39.88 45.7,39.12 v49.38,39.12 v60.81,39.12 61.32,38.61 65.38,38.61 65.76,38.99 v70.84,38.99 | 38.71,28.19 38.84,28.19 | 38.08,28.19 38.71,28.19 | 38.08,28.19 C30.1 36.93,27.69 38.08,26.54 | 40.36,23.11 40.36,23.62 39.09,23.62 38.84,23.62 | 38.71,23.62 38.84,23.62 | 38.71,23.62 C31.1 38.2,23.75 | 38.84,23.62 39.85,22.61 40.36,22.61 | 39.09,24.51 40.36,24.51 41.25,24.51 41.76,24 | v38.2,26.42 38.08,26.42 38.08,26.54 | 38.08,26.54 38.08,28.19 | 38.71,23.62 38.71,28.19 | v37.19,33.4 38.96,33.4 39.73,34.16 39.73,39.12 | v58.02,23.37 C67.2 | v51.54,22.1 R42.2 | v51.54,15.75 C65.2 | R48.2 67.92,15.75 C59.2 69.95,16 | VREF.P$1 69.95,20.32 | 69.95,20.32 69.95,16 | 69.95,20.32 v69.44,20.32 | 69.95,16 69.95,13.97 70.46,13.46 70.46,12.06 67.92,9.53 v66.65,9.53
  Top 1.27: v38.2,26.42 38.2,23.75 | TR3.1 55.22,9.53 TR1.2 v59.67,9.53 TR2.2 v66.65,9.53 | TR2.3 TR1.3
  Bottom 0.254: 50.9,11.3 51.41,10.79 51.41,6.99
  Bottom 0.356: 75.54,17.14 80.49,17.14
  Bottom 0.508: U5.10 21.57,39.62 21.31,39.88 | R37.2 52.05,40.26 U6.10 | 75.29,17.4 75.54,17.14 | 50.52,6.99 TR3_DIS.2 | R54.1 65.13,30.86 65.64,31.37 65.64,37.08 64.11,38.61 61.32,38.61 v60.81,39.12
  Bottom 1.016: R17.1 R18.2 81.13,9.14 81.13,16.51 80.49,17.14 | R36.2 21.31,39.88 v20.17,39.88 19.53,39.88 18.9,39.24 18.9,35.18 18.39,34.67 C47.2 R53.1 | v28.8,39.88 27.54,39.88 C46.2 | v60.81,39.12 59.67,40.26 C49.2 | R37.2 51.79,39.88 49.76,39.88 49.38,39.5 v49.38,39.12 49.38,35.05 48.87,34.54 C50.2 R55.1 C71.2 | C69.2 35.28,42.16 v35.28,39.12 | v38.2,26.42 37.19,27.43 37.19,30.86 | v37.19,33.4 37.19,30.86 | C67.2 v58.02,23.37 57.89,23.24 51.92,23.24 51.54,22.86 v51.54,22.1 v51.54,15.75 | v51.54,15.75 C60.2 53.06,15.49 R49.2 | 65.89,13.21 65.76,13.21 C68.2 | v69.44,20.32 68.56,20.32 R43.2 | VREF.P$1 72.37,20.32 75.29,17.4 | 50.9,11.3 50.9,15.11 v51.54,15.75 | v70.84,38.99 70.84,24.51 71.86,23.5 | 50.52,6.99 51.41,6.99 TR3.1 | 37.19,30.86 R8.1
  Bottom 1.27: 65.89,12.06 65.89,13.21 66.65,12.45 TR2.3 | TR2.3 65.89,11.3 | 65.89,9.53 65.89,11.3 | 65.89,9.53 v66.65,9.53 TR2.3 | 65.89,9.53 TR2.2 | 71.86,23.5 VREF.P$1 | TR2.3 65.89,12.06 | 65.89,11.3 65.89,12.06
VPP  (via drill 0.6)
  Top 0.508: v29.69,0.89 29.95,0.64 30.33,0.64 | 30.71,0.64 30.33,0.64 | 30.71,0.64 76.18,0.64 76.3,0.76 | v29.69,0.89 30.07,0.89 | 30.07,0.89 30.07,1.27 | 30.07,1.27 30.07,3.17 30.71,3.81 32.49,3.81 33.25,4.57 37.57,4.57 v38.08,5.08 | 30.07,0.89 30.33,0.64 | 30.07,1.27 30.71,0.64 | v29.69,0.89 30.07,1.27
  Top 0.762: 78.97,7.37 78.97,3.43 76.3,0.76 | C8.1 38.08,12.32 37.06,13.34 35.71,13.34 34.39,14.66 34.39,15.37 v34.27,15.37
  Top 1.016: C8.1 R1.1 38.08,9.78 v39.22,9.78 | v38.08,5.08 C72.1 | v34.27,15.37 C7.1
  Top 1.27: ICSP.2 81.38,18.92 81.38,9.78 78.97,7.37 | 33.12,19.81 v33.12,21.08 v34.39,21.08 33.12,19.81 | 33.12,19.81 L3.1
  Bottom 0.508: 36.42,9.78 33.59,6.95 U1.5 | v38.08,5.08 37.23,4.23 U1.38 | U1.17 36.42,14.73 36.04,15.11 34.52,15.11 v34.27,15.37
  Bottom 0.762: U3.8 26.52,3.05 27.03,2.54 C13.1 27.54,1.27 27.92,0.89 v29.69,0.89
  Bottom 1.016: C24.1 34.39,19.94 | 34.39,19.94 34.39,20.07 | 34.39,19.94 C25.1 | v38.08,5.08 38.08,9.78 | v34.27,15.37 33.38,16.26 33.38,17.02 | 38.08,9.78 v39.22,9.78 | 38.08,9.78 36.42,9.78
  Bottom 1.27: C26.+ 33.38,17.02 33.12,17.02 33.12,18.03 | 33.12,18.03 L2.2 | 33.12,18.03 C24.1 v33.12,21.08 v34.39,21.08 34.39,20.07

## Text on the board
tNames: + | 1 | + | + | + | 9 | 10 | Rev.B | MOD-EEG-SMT WWW.OLIMEX.COM (C) 2011
bNames: + | + | + | +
